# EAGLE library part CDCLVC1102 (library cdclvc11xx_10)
CDCLVC1102 3.3V and 2.5V LVCMOS High-Performance Clock Buffer - 1:2 Fan-out Source: http://www.ti.com/lit/ds/symlink/cdclvc1102.pdf
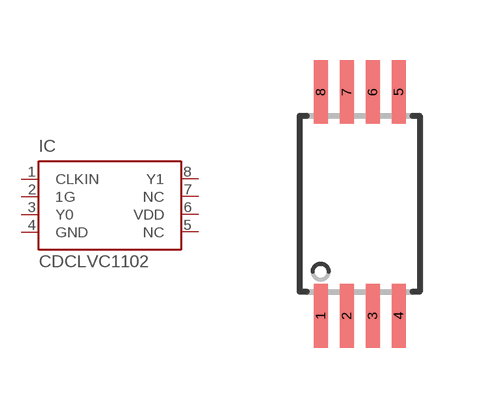
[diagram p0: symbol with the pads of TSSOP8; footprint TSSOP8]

Designator prefix IC

## CDCLVC1102PW (MF: Texas Instruments; MPN: CDCLVC1102; OC_FARNELL: 1829679; OC_NEWARK: 79R7906)  [TSSOP8]
1  CLKIN  in
2  1G  in
3  Y0  out
4  GND  pwr
5  NC  nc
6  VDD  pwr
7  NC  nc
8  Y1  out

## Footprint TSSOP8 (pad centres in mm)
TSSOP-8 Plastic Thin Srink Small Outline (PW) Source: http://www.ti.com/lit/ds/symlink/cdclvc1102.pdf
smd 0.35 x 1.6: 1 -0.975,-2.8; 2 -0.325,-2.8; 3 0.325,-2.8; 4 0.975,-2.8; 5 0.975,2.8; 6 0.325,2.8; 7 -0.325,2.8; 8 -0.975,2.8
